FUNCTION_BLOCK FB_CountEX EXTENDS FB_Count
VAR_INPUT
END_VAR
VAR_OUTPUT
END_VAR
VAR
END_VAR

METHOD M_Check : BOOL
VAR_INPUT
	bCheckValue: BOOL;
END_VAR
IF bCheckValue THEN
	IF i=k THEN
		M_Check:=TRUE;
	ELSE
		M_Check:=FALSE;
	END_IF  
END_IF
END_METHOD

END_FUNCTION_BLOCK
